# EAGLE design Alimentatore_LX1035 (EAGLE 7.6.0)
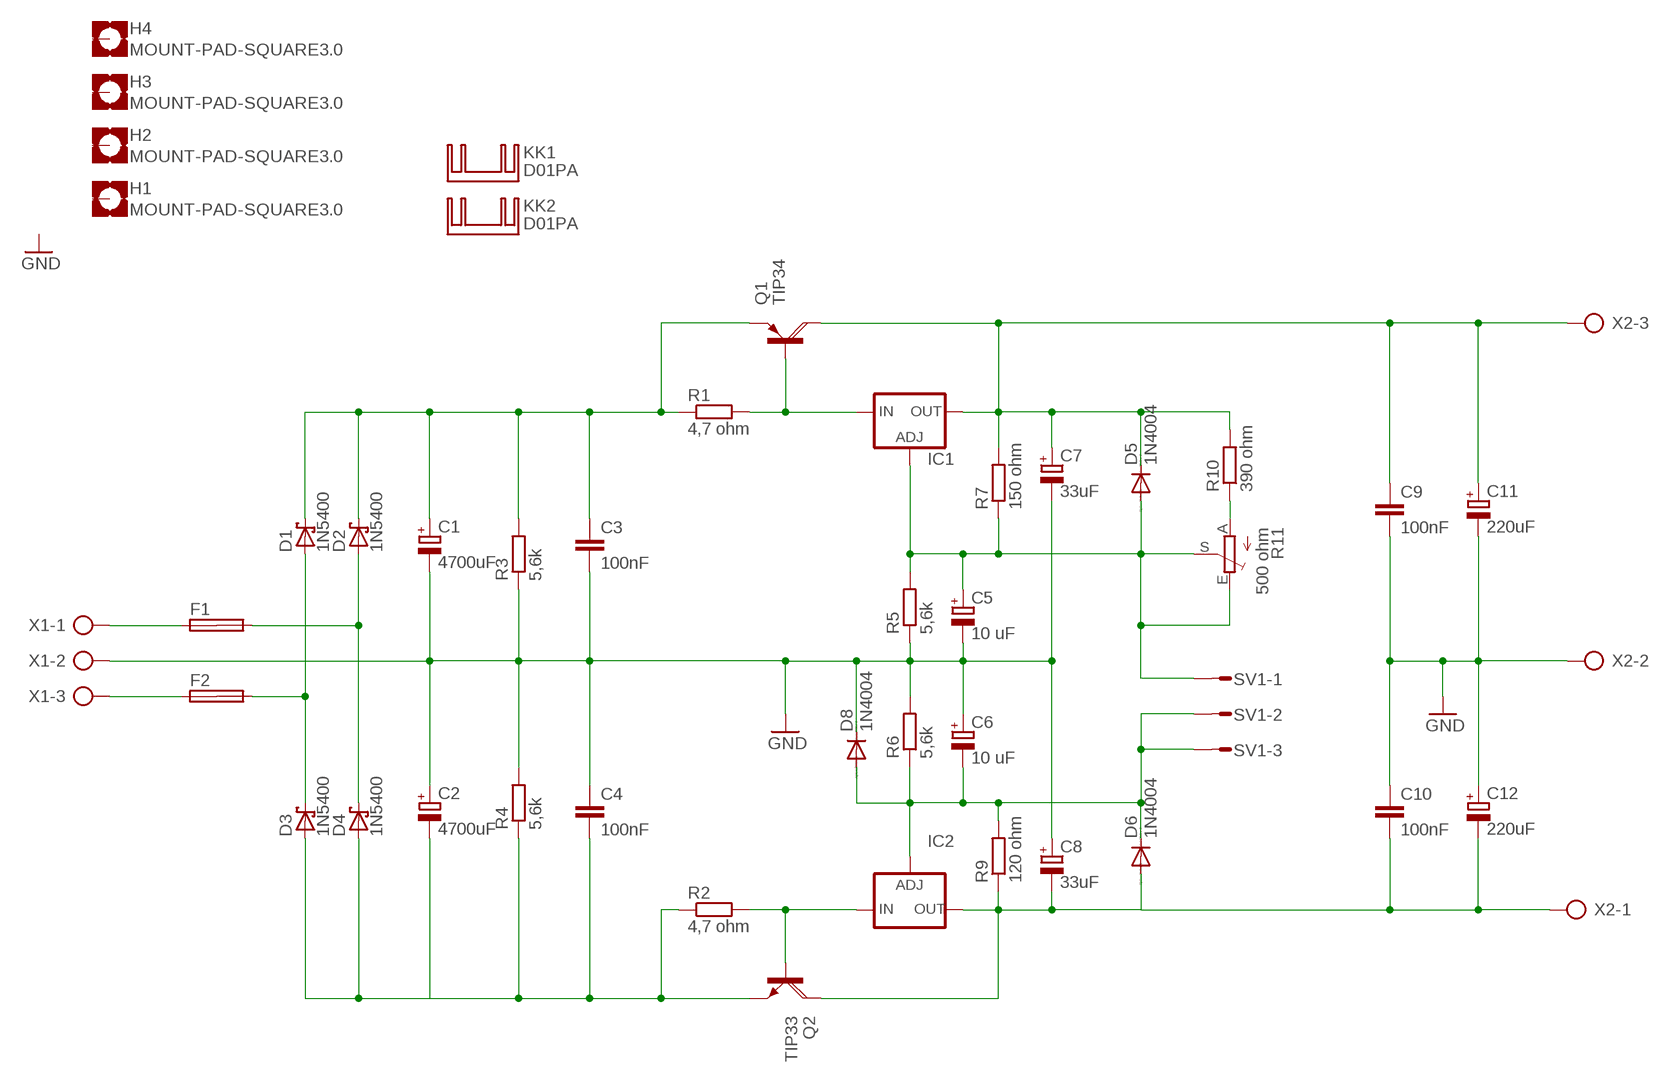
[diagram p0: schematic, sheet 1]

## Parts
C1  4700uF  CPOL-EUE10-20  [EB20D]
C2  4700uF  CPOL-EUE10-20  [EB20D]
C3  100nF  C-EU102-043X133  [C102-043X133]
C4  100nF  C-EU102-043X133  [C102-043X133]
C5  10 uF  CPOL-EUE2.5-7  [E2,5-7]
C6  10 uF  CPOL-EUE2.5-7  [E2,5-7]
C7  33uF  CPOL-EUE5-10.5  [E5-10,5]
C8  33uF  CPOL-EUE5-10.5  [E5-10,5]
C9  100nF  C-EU050-025X075  [C050-025X075]
C10  100nF  C-EU050-025X075  [C050-025X075]
C11  220uF  CPOL-EUE5-10.5  [E5-10,5]
C12  220uF  CPOL-EUE5-10.5  [E5-10,5]
D1  1N5400  15KEXX  [CB429-17]
D2  1N5400  15KEXX  [CB429-17]
D3  1N5400  15KEXX  [CB429-17]
D4  1N5400  15KEXX  [CB429-17]
D5  1N4004  [DO41-10]
D6  1N4004  [DO41-10]
D8  1N4004  [DO41-10]
F1  SHK20L  [SHK20L]
F2  SHK20L  [SHK20L]
H1  MOUNT-PAD-SQUARE3.0  [3,0-PAD-SQUARE]
H2  MOUNT-PAD-SQUARE3.0  [3,0-PAD-SQUARE]
H3  MOUNT-PAD-SQUARE3.0  [3,0-PAD-SQUARE]
H4  MOUNT-PAD-SQUARE3.0  [3,0-PAD-SQUARE]
IC1  LM317TS  [317TS]
IC2  LM337TS  [337TS]
KK1  D01PA  [D01PA]
KK2  D01PA  [D01PA]
Q1  TIP34  TIP147  [SOT93]
Q2  TIP33  TIP142  [SOT93]
R1  4,7 ohm  R-EU_0411/15  [0411/15]
R2  4,7 ohm  R-EU_0411/15  [0411/15]
R3  5,6k  R-EU_0207/10  [0207/10]
R4  5,6k  R-EU_0207/10  [0207/10]
R5  5,6k  R-EU_0207/10  [0207/10]
R6  5,6k  R-EU_0207/10  [0207/10]
R7  150 ohm  R-EU_0207/10  [0207/10]
R9  120 ohm  R-EU_0207/10  [0207/10]
R10  390 ohm  R-EU_0207/10  [0207/10]
R11  500 ohm  TRIM_EU-CA9V  [CA9V]
SV1  S03P  [S03P]
X1  AK500/3-H  [AK500/3-H]
X2  AK500/3-H  [AK500/3-H]

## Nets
GND: C1.- C2.+ C3.2 C4.1 C5.- C6.+ C7.- C8.+ C9.2 C10.1 C11.- C12.+ D8.C R3.1 R4.2 R5.1 R6.2 X1.2 X2.2
N$1: C7.+ C9.1 C11.+ D5.C IC1.2(OUT) Q1.C R7.2 R10.2 X2.3
N$2: C5.+ D5.A IC1.1(ADJ) R5.2 R7.1 R11.E R11.S SV1.1
N$3: IC1.3(IN) Q1.B R1.2
N$4: R10.1 R11.A
N$5: C8.- C10.2 C12.- D6.A IC2.3(OUT) Q2.C R9.1 X2.1
N$6: IC2.2(IN) Q2.B R2.2
N$8: C1.+ C3.1 D1.C D2.C Q1.E R1.1 R3.2
N$9: C6.- D6.C D8.A IC2.1(ADJ) R6.1 R9.2 SV1.2 SV1.3
N$10: C2.- C4.2 D3.A D4.A Q2.E R2.1 R4.1
N$11: D1.A D3.C F2.2A
N$12: D2.A D4.C F1.2A
N$14: F2.1A X1.3
N$15: F1.1A X1.1
Unconnected: F1.1B F1.2B F2.1B F2.2B H1.B3,0(MOUNT) H2.B3,0(MOUNT) H3.B3,0(MOUNT) H4.B3,0(MOUNT)

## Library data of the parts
C1 C2 C5-C8 C11 C12 = rcl:CPOL-EU: POLARIZED CAPACITOR, European symbol
C3 C4 C9 C10 = rcl:C-EU: CAPACITOR, European symbol
D1-D4 = diode:15KEXX: DIODE
D5 D6 D8 = diode:1N4004: DIODE
F1 F2 = fuse:SHK20L: FUSE HOLDER 5 x 20 mm, SH contact, SHH1 Schukat, E1073 Buerklin; OC_FARNELL: unknown; OC_NEWARK: unknown
H1-H4 = holes:MOUNT-PAD-SQUARE: MOUNTING PAD, square
IC1 = v-reg:LM317TS: VOLTAGE REGULATOR
IC2 = v-reg:LM337TS: VOLTAGE REGULATOR
KK1 KK2 = heatsink:D01PA: HEATSINK
Q1 = transistor-power:TIP147: PNP DARLINGTON TRANSISTOR
Q2 = transistor-power:TIP142: NPN DARLINGTON TRANSISTOR
R1-R7 R9 R10 = rcl:R-EU_: RESISTOR, European symbol
R11 = pot:TRIM_EU-: POTENTIOMETER
SV1 = con-amp-mt:S03P: AMP MT CONNECTOR; OC_FARNELL: unknown; OC_NEWARK: unknown
X1 X2 = con-ptr500:AK500/3-H: CONNECTOR Aug. 2004 / PTR Meßtechnik: Die Bezeichnung der Serie AK505 wurde geändert. Es handelt sich hierbei um AK500 in horizontaler Ausführung.; OC_FARNELL: unknown; OC_NEWARK: unknown

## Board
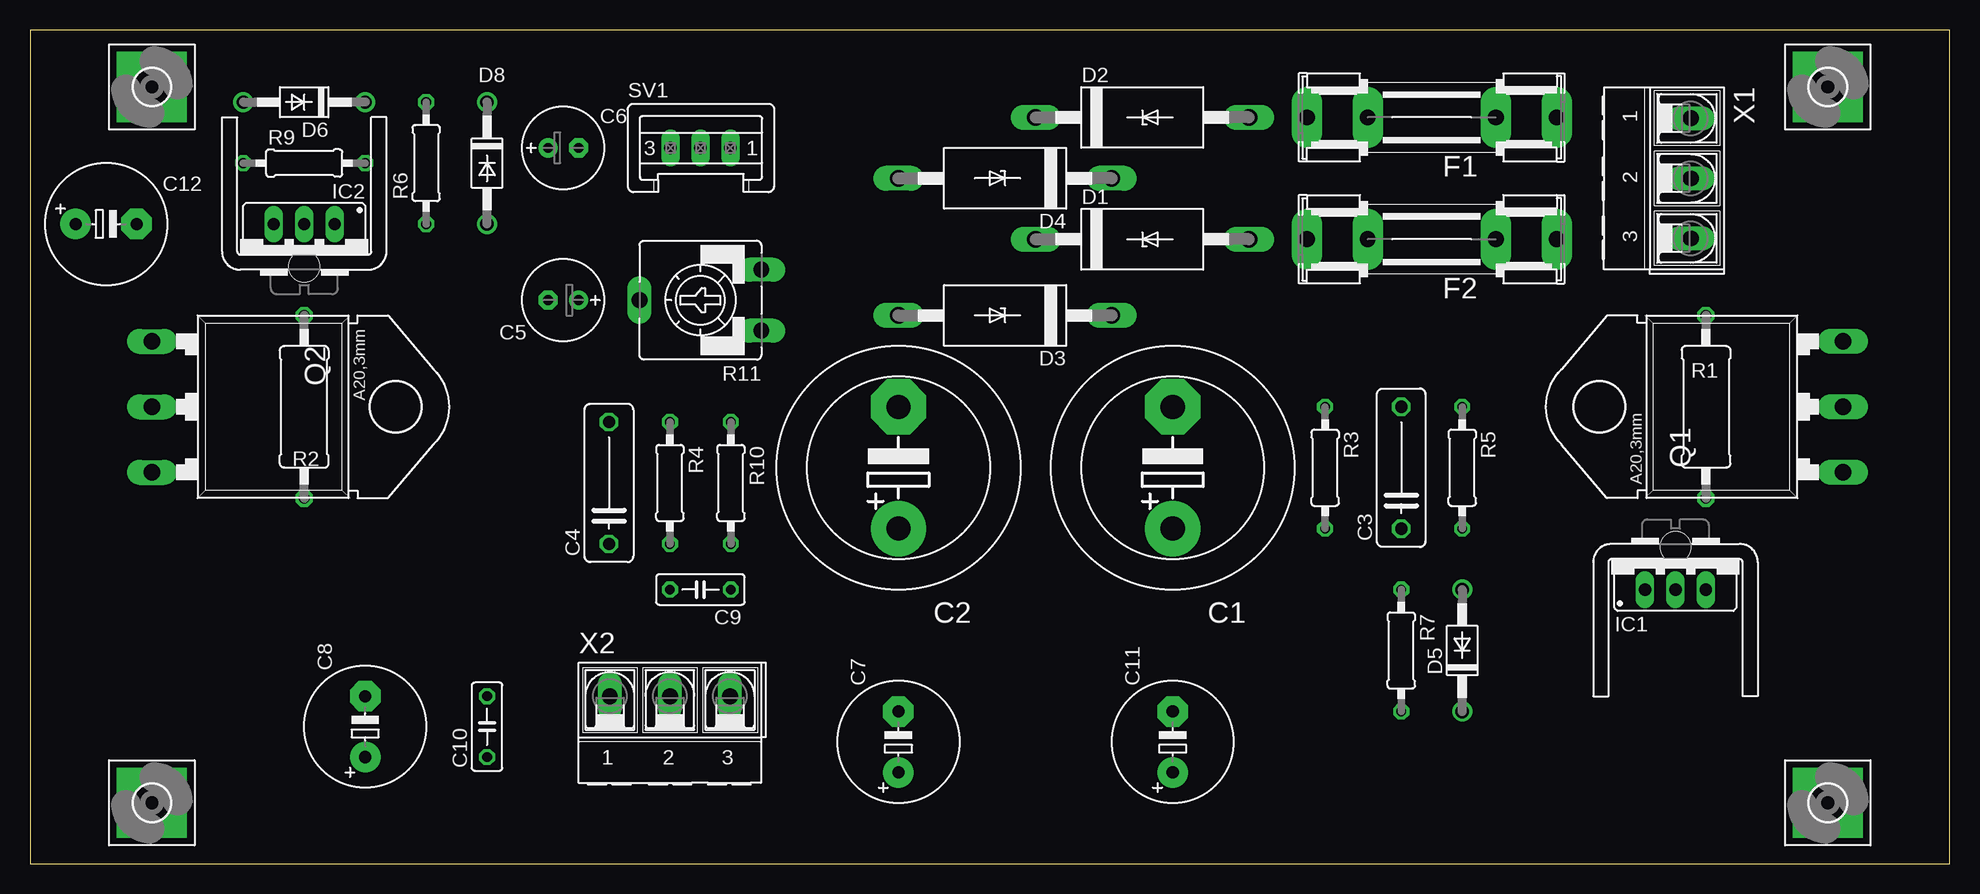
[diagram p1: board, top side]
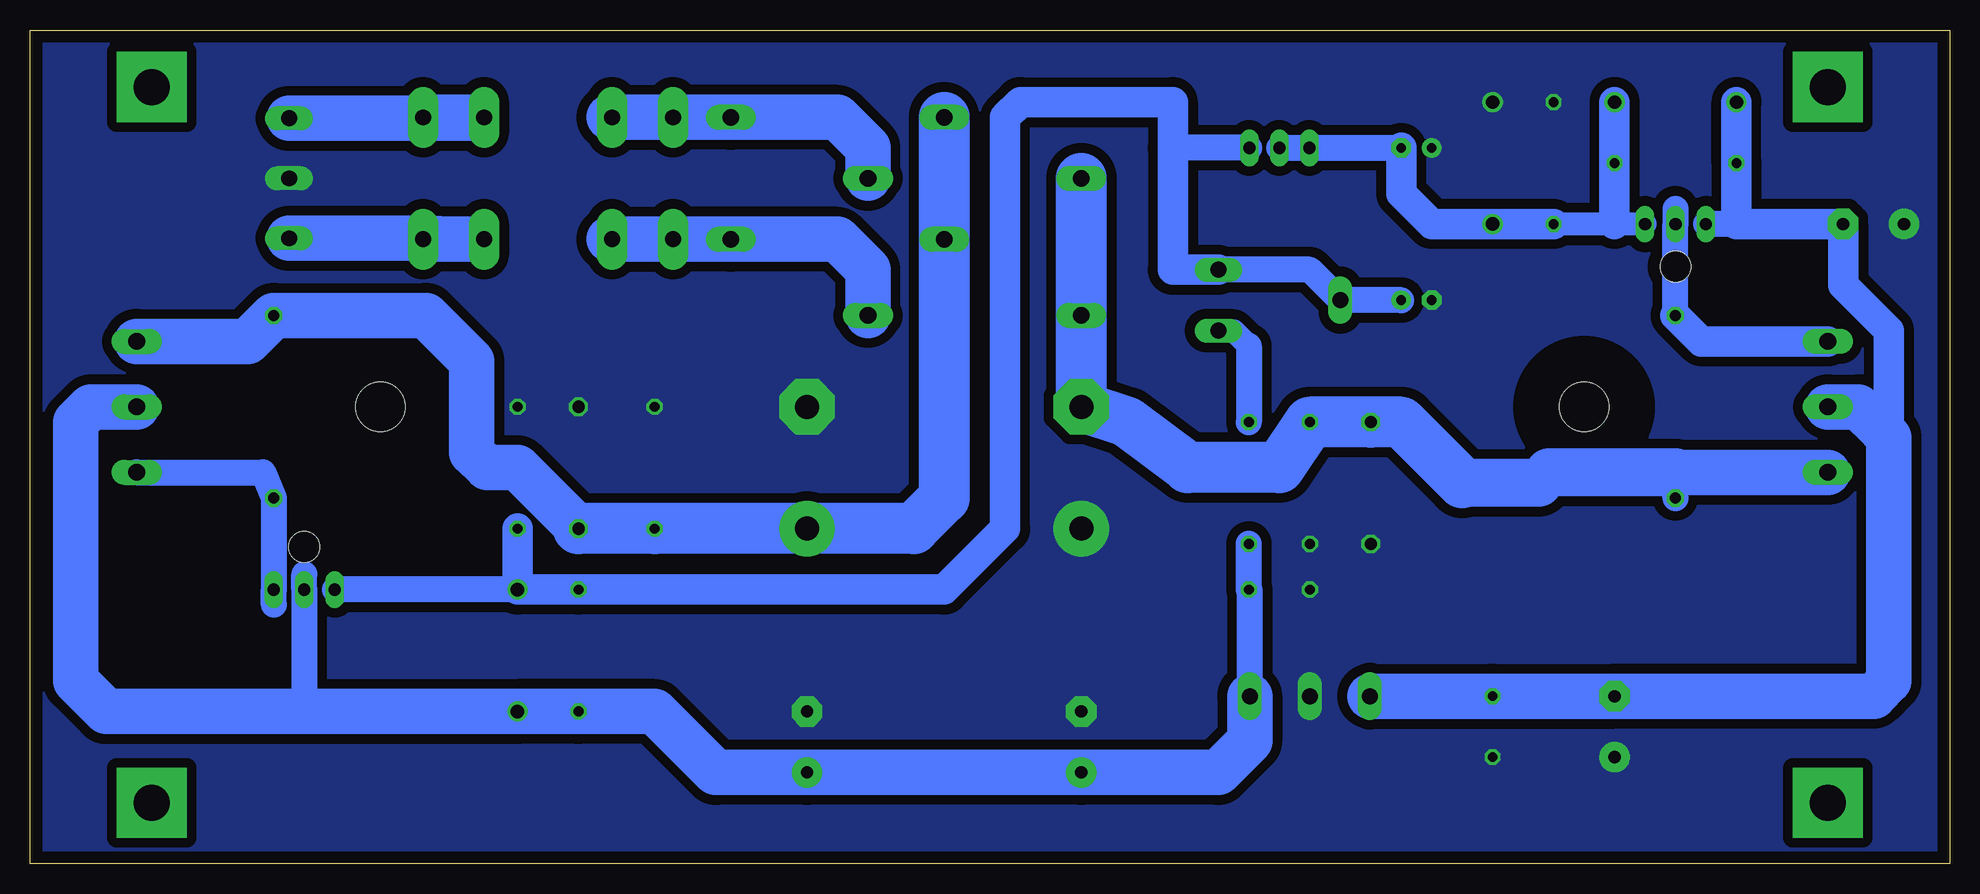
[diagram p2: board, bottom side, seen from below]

Size 160 x 69.52 mm. Coordinates in mm from the lower left corner, seen from the top.
Outline: 0,0 160,0 160,69.52 0,69.52 0,0
Copper layers (1*16): Top 0.035mm / dielectric 1.5mm / Bottom 0.035mm
Design rules "default *": minimum track width 10mil, minimum drill 24mil, track to track 8mil, track to pad 8mil, pad to pad 8mil, via to via 8mil, smd to smd 8mil, copper to edge 40mil, drill to drill 8mil, minimum pad ring 10mil, minimum via ring 8mil, stop-mask expansion 4mil, vias tented up to drill 0mil, thermal gap 0mil

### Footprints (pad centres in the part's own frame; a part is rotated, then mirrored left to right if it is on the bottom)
EB20D = drill 2.007 pad 4.597: + -5.08,0 | drill 2.007 pad 4.597 octagon: - 5.08,0
C102-043X133 = drill 1.016 octagon: 1 -5.08,0; 2 5.08,0
E2,5-7 = drill 0.813 pad 1.6: + -1.27,0 | drill 0.813 pad 1.6 octagon: - 1.27,0
E5-10,5 = drill 1.016 pad 2.54: + -2.54,0 | drill 1.016 pad 2.54 octagon: - 2.54,0
C050-025X075 = drill 0.813 octagon: 1 -2.54,0; 2 2.54,0
CB429-17 = drill 1.397 long: A 8.89,0; C -8.89,0
DO41-10 = drill 1.118: A 5.08,0; C -5.08,0
SHK20L = drill 1.321 pad 2.54 long: 1A -10.414,0; 1B -5.334,0; 2A 10.414,0; 2B 5.334,0
3,0-PAD-SQUARE = drill 3 pad 5.842 square: B3,0 0,0
317TS = drill 1.016 long: 1 -2.54,-2.54; 2 0,-2.54; 3 2.54,-2.54
337TS = drill 1.016 long: 1 -2.54,-2.54; 2 0,-2.54; 3 2.54,-2.54
D01PA = hole 2.54: 0,-1.016
SOT93 = drill 1.397 long: B -5.461,-10.16; C 0,-10.16; E 5.461,-10.16 | hole 4.115: 0,10.16
0411/15 = drill 0.914 octagon: 1 -7.62,0; 2 7.62,0
0207/10 = drill 0.813 octagon: 1 -5.08,0; 2 5.08,0
CA9V = drill 1.321 long: A -2.54,-5.08; E 2.54,-5.08; S 0,5.08
S03P = drill 1.016 long: 1 2.5,0; 2 0,0; 3 -2.5,0
AK500/3-H = drill 1.321 long: 1 -5.004,0; 2 0,0; 3 5.004,0

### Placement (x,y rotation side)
C1  95.25,33.02 90 top
C2  72.39,33.02 90 top
C3  114.3,33.02 90 top
C4  48.26,31.75 90 top
C5  44.45,46.99 180 top
C6  44.45,59.69 0 top
C7  72.39,10.16 90 top
C8  27.94,11.43 90 top
C9  55.88,22.86 180 top
C10  38.1,11.43 90 top
C11  95.25,10.16 90 top
C12  6.35,53.34 0 top
D1  92.71,52.07 0 top
D2  92.71,62.23 0 top
D3  81.28,45.72 180 top
D4  81.28,57.15 180 top
D5  119.38,17.78 90 top
D6  22.86,63.5 180 top
D8  38.1,58.42 270 top
F1  116.84,62.23 180 top
F2  116.84,52.07 180 top
H1  10.16,64.77 0 top
H2  10.16,5.08 0 top
H3  149.86,5.08 0 top
H4  149.86,64.77 0 top
IC1  137.16,25.4 0 top
IC2  22.86,50.8 180 top
KK1  22.86,50.8 0 top
KK2  137.16,25.4 180 top
Q1  140.97,38.1 90 top
Q2  20.32,38.1 270 top
R1  139.7,38.1 270 top
R2  22.86,38.1 90 top
R3  107.95,33.02 270 top
R4  53.34,31.75 270 top
R5  119.38,33.02 270 top
R6  33.02,58.42 90 top
R7  114.3,17.78 270 top
R9  22.86,58.42 0 top
R10  58.42,31.75 270 top
R11  55.88,46.99 90 top
SV1  55.88,59.69 0 top
X1  138.43,57.15 270 top
X2  53.34,13.97 0 top

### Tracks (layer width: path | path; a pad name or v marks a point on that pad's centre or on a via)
GND
  pour Bottom (isolate 0.813): 0,69.85 160.02,69.85 160.02,0 0,0
N$1
  Bottom 1.676: 58.34,22.78 C9.1
  Bottom 2.184: X2.3 58.34,22.78 | C9.1 R10.2 | 137.16,24.13 IC1.2 137.16,12.7
  Bottom 3.81: X2.3 58.34,10.24 60.96,7.62 C7.+ C11.+ 102.87,7.62 107.95,12.7 R7.2 D5.C 137.16,12.7 153.67,12.7 156.21,15.24 156.21,36.83 154.94,38.1 Q1.C
N$2
  Bottom 2.184: R11.E 53.34,49.53 R11.S C5.+ | SV1.1 64.77,59.69 | D5.A IC1.1
  Bottom 2.54: R11.E 64.77,49.53 64.77,59.69 64.77,63.5 77.47,63.5 78.74,62.23 78.74,27.94 83.82,22.86 R7.1 D5.A R5.2
N$3
  Bottom 2.184: Q1.B 140.59,32.64 R1.2 IC1.3 139.7,21.59
N$4
  Bottom 1.93: R11.A 59.69,44.45 58.42,43.18
  Bottom 2.184: 58.42,43.18 R10.1
N$5
  Bottom 1.93: 5.08,36.83 5.71,36.2
  Bottom 2.184: 17.78,53.34 IC2.3
  Bottom 2.54: D6.A R9.1 17.78,53.34 C12.- 8.89,48.26 5.08,44.45 5.08,36.83
  Bottom 3.81: X2.1 C10.2 C8.- 6.35,13.97 5.08,15.24 5.08,35.56 5.71,36.2 7.62,38.1 Q2.C
N$6
  Bottom 2.184: R2.2 IC2.2 22.86,54.61
  Bottom 2.54: Q2.B 20.7,43.56 R2.2
N$8
  Bottom 3.81: Q1.E 141.86,43.56 R1.1 127,45.72 123.19,41.91 123.19,34.29 121.92,33.02 119.38,33.02 C3.1
  Bottom 4.25: D2.C D1.C 83.82,30.48 86.36,27.94 C1.+ R3.2 C3.1
N$9
  Bottom 1.93: IC2.1 27.94,53.34 R6.1
  Bottom 2.184: SV1.3 SV1.2 C6.-
  Bottom 2.54: R6.1 D8.A 43.18,53.34 45.72,55.88 C6.- | D6.C R9.2 27.94,53.34
N$10
  Bottom 2.184: R2.1 22.86,32.64
  Bottom 2.54: 33.4,32.64 34.29,31.75
  Bottom 3.81: Q2.E 22.86,32.64
  Bottom 4: 22.86,32.64 33.4,32.64 | 34.29,31.75 40.64,31.75
  Bottom 4.25: D4.A D3.A C2.- 68.58,36.83 63.5,33.02 55.88,33.02 R4.1 C4.2 45.72,36.83 40.64,31.75
N$11
  Bottom 3.81: D3.C 90.17,49.53 92.71,52.07 D1.A F2.2A 111.76,52.07
N$12
  Bottom 3.81: D4.C 90.17,59.69 92.71,62.23 D2.A F1.2A 111.76,62.23
N$14
  Bottom 3.81: X1.3 128.27,52.15 123.19,52.07 F2.1A
N$15
  Bottom 3.81: X1.1 123.19,62.15 123.19,62.23 F1.1A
